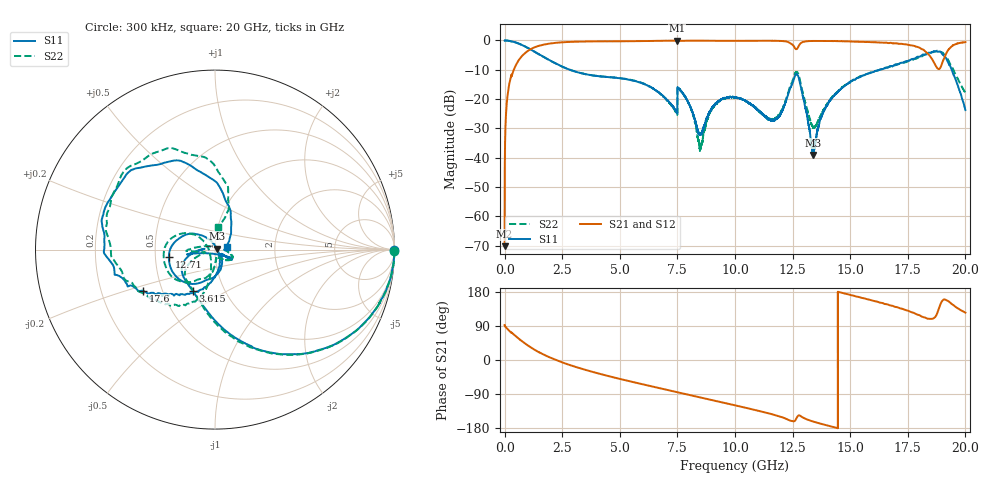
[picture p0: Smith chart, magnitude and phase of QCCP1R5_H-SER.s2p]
!{QCCP1R5}
!Johanson Technology Inc.
!www.johansontechnology.com
!Test Board Conditions:
!Substrate Type  RO4350B
!Substrate Thickness  20 mil
!Substrate Dk  3.66
!TL Type: GCPW
!TL Trace Width  36 mil
!TL Gap  12 mil
!Electrode orientation  Horizontal
!DUT TOPOLOGY	SERIES
!Mounting Pad LxW  26x36 mil
! Created Sat Jan  9 18:25:21 2021
# hz S ma R 50
! 2 Port Network Data from SP1.SP block
! freq  magS11  angS11  magS21  angS21  magS12  angS12  magS22  angS22
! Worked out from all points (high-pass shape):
!   20001 points, 300 kHz to 20 GHz, reference 50 ohm
!   highest |S21| = -0.06 dB at 7.479 GHz (marker M1); lowest = -70.1 dB at 300 kHz (marker M2)
!   |S21| within 3 dB of the highest: 1.117 GHz to 18.14 GHz (17.03 GHz wide, 177 % of centre); 19.27 GHz to end of sweep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
!   lowest |S11| = -39.1 dB at 13.4 GHz (marker M3), VSWR 1.02, Z = 51 + j0.59 ohm
!   |S11| at or under -10 dB: 2.838065 GHz to 2.838639 GHz (574 kHz wide, 0.0202 % of centre); 2.84 GHz to 16.28 GHz (13.44 GHz wide, 141 % of centre); 19.41 GHz to end of sweep
!   |S22| runs from -37.7 to 0.0 dB; largest |S21 - S12| = 0.014
!   S11 on the Smith chart (normalised r, x): 300 kHz: open; 3.615 GHz: 0.71, -0.35; 12.71 GHz: 0.59, -0.05; 17.6 GHz: 0.39, -0.23; 20 GHz: 1.14, +0.03
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300000  0.9951 -0.3  0.0003109 92.4  0.0003137 97.6  0.997 -0.3
1.363e8  0.992 -8.4  0.1225 81.2  0.1227 81.3  0.9917 -8.5
5.143e8  0.9155 -28.3  0.3974 61.3  0.3972 61.3  0.9157 -28.4
1.7593e9  0.5075 -76.7  0.8571 12.5  0.8587 12.5  0.5064 -77.8
3.3343e9  0.2761 -112.9  0.9575 -22.9  0.9569 -22.9  0.2763 -112.6
3.6153e9  0.262 -118.3  0.9614 -27.9  0.9615 -27.8  0.2615 -116.9
6.6673e9  0.1323 -169.9  0.9855 -73.5  0.9861 -73.5  0.1312 -156.0
7.4793e9  0.05881 176.5  0.9929 -84.7  0.9921 -84.7  0.05631 -164.1
7.8803e9  0.1023 -168.4  0.9888 -90.4  0.9888 -90.4  0.1022 172.8
8.5003e9  0.02505 -91.6  0.9909 -99.0  0.9914 -98.9  0.01417 74.6
9.0733e9  0.07591 -29.2  0.9881 -106.8  0.9876 -106.8  0.0727 -9.0
1.00003e10  0.1062 -31.5  0.9851 -119.6  0.9858 -119.6  0.1071 -29.6
1.16393e10  0.04375 -33.6  0.9866 -143.7  0.9876 -143.7  0.04507 -76.2
1.27123e10  0.2608 -170.7  0.7371 -149.2  0.7373 -149.0  0.2861 -177.4
1.33343e10  0.01529 64.0  0.9768 -161.3  0.9778 -161.3  0.03618 173.3
1.33973e10  0.01113 31.3  0.981 -162.5  0.9803 -162.5  0.03319 -172.4
1.42903e10  0.114 -80.8  0.977 -177.3  0.9778 -177.3  0.1151 -100.6
1.66673e10  0.3515 -135.3  0.9008 145.6  0.9042 145.3  0.351 -118.4
1.76003e10  0.4612 -150.2  0.8297 127.6  0.832 127.3  0.4521 -143.7
1.85103e10  0.6197 173.8  0.5079 108.7  0.503 108.4  0.6227 165.7
1.89923e10  0.5929 128.0  0.4105 155.9  0.4075 156.3  0.6259 116.2
2e10  0.06521 12.6  0.9359 125.1  0.934 125.1  0.1285 82.6
